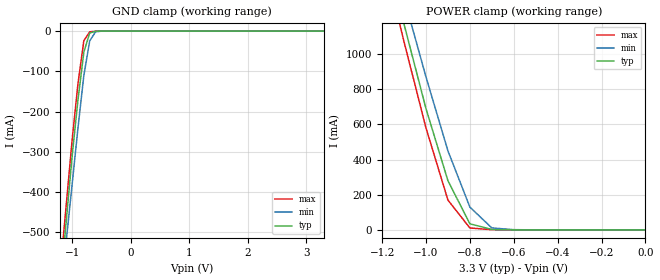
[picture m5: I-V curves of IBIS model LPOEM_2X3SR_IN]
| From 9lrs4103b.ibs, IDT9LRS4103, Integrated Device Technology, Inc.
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|   Model LPOEM_2X3SR_IN
[Model]   LPOEM_2X3SR_IN
Model_type   Input
Enable   Active-High
Vinl =   0.80V
Vinh =   2.00V
C_comp   3.40pF   2.85pF   3.95pF
[Temperature Range]   27.00   70.00   0.000
[Voltage Range]   3.30V   3.00V   3.70V
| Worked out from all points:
|   GND clamp passes 1 mA (typ) near -0.61 V on its own axis
|   POWER clamp passes 1 mA (typ) near -0.61 V on its own axis
[GND_clamp]
| voltage   I(typ)   I(min)   I(max)
-3.3V     -4.16A     -4.01A     -4.26A
-1.2V     -630mA     -670mA     -590mA
-1.1V     -470mA     -520mA     -430mA
-1V       -310mA     -380mA     -270mA
-900mV    -170mA     -240mA     -130mA
-800mV    -52.15mA   -110mA     -23.62mA
-700mV    -4.69mA    -24.32mA   -1.84mA
-600mV    -430uA     -1.9mA     -210uA
-500mV    -36.28uA   -150uA     -14.75uA
3.3V      1.51nA     23.36uA    830pA
[POWER_clamp]
| voltage   I(typ)   I(min)   I(max)
-3.3V     12.9A      12.41A     13.22A
-1.2V     1.67A      1.79A      1.58A
-1.1V     1.17A      1.32A      1.07A
-1V       690mA      870mA      580mA
-900mV    280mA      450mA      170mA
-800mV    35.15mA    130mA      11.29mA
-700mV    2.74mA     11.68mA    1.47mA
-600mV    740uA      1.69mA     420uA
0V        1.51nA     1.44nA     1.69nA
